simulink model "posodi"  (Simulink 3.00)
settings: Solver=ode45  StartTime=0.0  StopTime=1200  RelTol=1e-3
undefined symbols (not defined in the file or in its folder): dec2bin, H10_X1, H10_X2, H12_X1, H12_X2, H7_X1, H7_X2, H8_X1, H8_X2, sgn
libraries: simulink3 x1

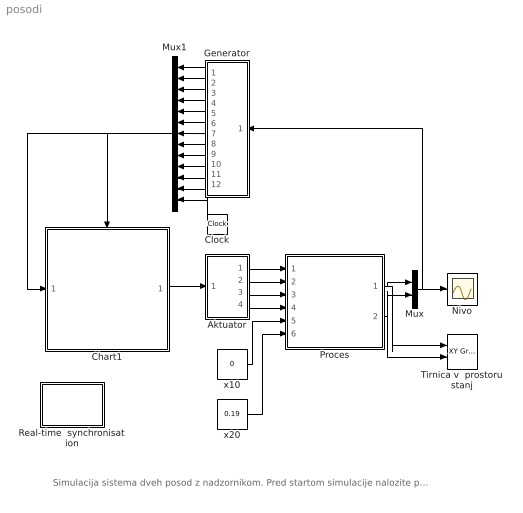
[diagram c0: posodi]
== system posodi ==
  note: Simulacija sistema dveh posod z nadzornikom. Pred startom simulacije nalozite podatke z ukazom "load meje".
  Aktuator : Subsystem
  Chart1 : Stateflow chart
  Clock : Clock
  Generator : Subsystem  Orientation=left
  Mux : Mux  Inputs=2
  Mux1 : Mux  Orientation=left  Inputs=13
  Nivo : Scope
  Proces : Subsystem
  Real-time  synchronisation : Subsystem  mask(Real-time synchronisation){ts=10, tf=20}
      mask prompts: ts "Sample time"; tf "Scale factor"
      mask help: Real-time synchronisation block
  Tirnica v  prostoru stanj : simulink3/Sinks/XY Graph  xmin=0  xmax=1.4  ymin=0  ymax=1.4  st=-1
  x10 : Constant  Value=0
  x20 : Constant  Value=0.19
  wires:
  Aktuator/1(u1) -> Proces/1(u1)
  Aktuator/2(u2) -> Proces/2(u2)
  Aktuator/3(u3) -> Proces/3(u3)
  Aktuator/4(u4) -> Proces/4(u4)
  Chart1/1(u) -> Aktuator/1(us)
  Proces/1(x1) -> Mux/1, Tirnica v  prostoru stanj/1
  Proces/2(x2) -> Mux/2, Tirnica v  prostoru stanj/2
  Mux/1 -> Nivo/1, Generator/1(x)
  Mux1/1 -> Chart1/Trigger, Chart1/1(h)
  x10/1 -> Proces/5(x10)
  x20/1 -> Proces/6(x20)
  Generator/1(h1) -> Mux1/1
  Generator/2(h2) -> Mux1/2
  Generator/3(h3) -> Mux1/3
  Generator/4(h4) -> Mux1/4
  Generator/5(h5) -> Mux1/5
  Generator/6(h6) -> Mux1/6
  Generator/7(h7) -> Mux1/7
  Generator/8(h8) -> Mux1/8
  Generator/9(h9) -> Mux1/9
  Generator/10(h10) -> Mux1/10
  Generator/11(h11) -> Mux1/11
  Generator/12(h12) -> Mux1/12
  Clock/1 -> Mux1/13

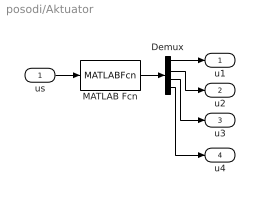
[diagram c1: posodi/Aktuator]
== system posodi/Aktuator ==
  us : Inport  Port=1  PortWidth=-1  SampleTime=-1  DataType=auto
  Demux : Demux  Outputs=4
  MATLAB Fcn : MATLABFcn  MATLABFcn=str2num(dec2bin(u(1)-1,4)')  OutputWidth=-1  OutputSignalType=auto
  u1 : Outport  Port=1
  u2 : Outport  Port=2
  u3 : Outport  Port=3
  u4 : Outport  Port=4
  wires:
  MATLAB Fcn/1 -> Demux/1
  Demux/1 -> u1/1
  Demux/2 -> u2/1
  us/1 -> MATLAB Fcn/1
  Demux/3 -> u3/1
  Demux/4 -> u4/1

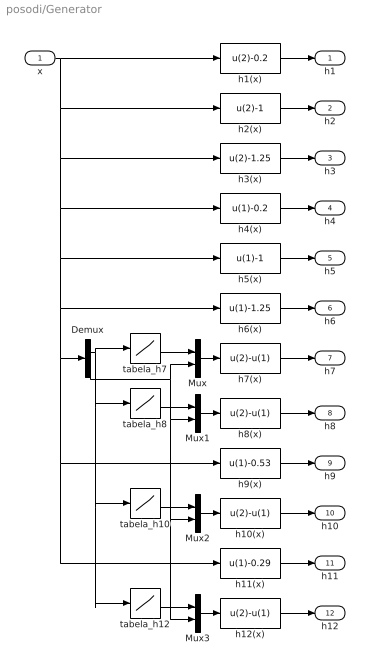
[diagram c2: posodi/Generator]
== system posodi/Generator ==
  x : Inport  Port=1  PortWidth=-1  SampleTime=-1  DataType=auto
  Demux : Demux  Outputs=2
  Mux{,1..3} (4 alike) : Mux  Inputs=2
  h1(x) : Fcn  Expr=u(2)-0.2
  h10(x) : Fcn  Expr=u(2)-u(1)
  h11(x) : Fcn  Expr=u(1)-0.29
  h12(x) : Fcn  Expr=u(2)-u(1)
  h2(x) : Fcn  Expr=u(2)-1
  h3(x) : Fcn  Expr=u(2)-1.25
  h4(x) : Fcn  Expr=u(1)-0.2
  h5(x) : Fcn  Expr=u(1)-1
  h6(x) : Fcn  Expr=u(1)-1.25
  h7(x) : Fcn  Expr=u(2)-u(1)
  h8(x) : Fcn  Expr=u(2)-u(1)
  h9(x) : Fcn  Expr=u(1)-0.53
  tabela_h10 : Lookup  InputValues=H10_X1  OutputValues=H10_X2
  tabela_h12 : Lookup  InputValues=H12_X1  OutputValues=H12_X2
  tabela_h7 : Lookup  InputValues=H7_X1  OutputValues=H7_X2
  tabela_h8 : Lookup  InputValues=H8_X1  OutputValues=H8_X2
  h1 : Outport  Port=1
  h2 : Outport  Port=2
  h3 : Outport  Port=3
  h4 : Outport  Port=4
  h5 : Outport  Port=5
  h6 : Outport  Port=6
  h7 : Outport  Port=7
  h8 : Outport  Port=8
  h9 : Outport  Port=9
  h10 : Outport  Port=10
  h11 : Outport  Port=11
  h12 : Outport  Port=12
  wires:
  x/1 -> h1(x)/1, h2(x)/1, h4(x)/1, h5(x)/1, h9(x)/1, h11(x)/1, Demux/1, h6(x)/1, h3(x)/1
  h1(x)/1 -> h1/1
  h4(x)/1 -> h4/1
  h9(x)/1 -> h9/1
  h11(x)/1 -> h11/1
  Demux/1 -> tabela_h7/1, tabela_h8/1, tabela_h10/1, tabela_h12/1
  tabela_h7/1 -> Mux/1
  Mux/1 -> h7(x)/1
  h7(x)/1 -> h7/1
  Mux1/1 -> h8(x)/1
  h8(x)/1 -> h8/1
  tabela_h8/1 -> Mux1/1
  Mux2/1 -> h10(x)/1
  h10(x)/1 -> h10/1
  Mux3/1 -> h12(x)/1
  h12(x)/1 -> h12/1
  tabela_h10/1 -> Mux2/1
  tabela_h12/1 -> Mux3/1
  h2(x)/1 -> h2/1
  h3(x)/1 -> h3/1
  h5(x)/1 -> h5/1
  h6(x)/1 -> h6/1
  Demux/2 -> Mux1/2, Mux2/2, Mux3/2, Mux/2

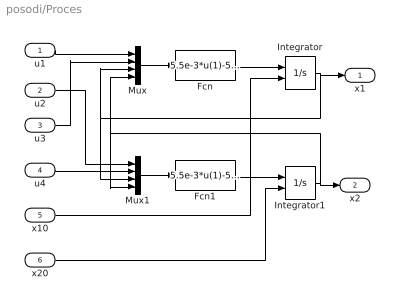
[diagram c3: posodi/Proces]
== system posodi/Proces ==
  u1 : Inport  Port=1  PortWidth=-1  SampleTime=-1  DataType=auto
  u2 : Inport  Port=2  PortWidth=-1  SampleTime=-1  DataType=auto
  u3 : Inport  Port=3  PortWidth=-1  SampleTime=-1  DataType=auto
  u4 : Inport  Port=4  PortWidth=-1  SampleTime=-1  DataType=auto
  x10 : Inport  Port=5  PortWidth=-1  SampleTime=-1  DataType=auto
  x20 : Inport  Port=6  PortWidth=-1  SampleTime=-1  DataType=auto
  Fcn : Fcn  Expr=5.5e-3*u(1)-5e-3*sqrt(u(3))*u(2)-2e-3*sgn(u(3)-u(4))*sqrt(abs(u(3)-u(4)))
  Fcn1 : Fcn  Expr=5.5e-3*u(1)-5e-3*sqrt(u(4))*u(2)+2e-3*sgn(u(3)-u(4))*sqrt(abs(u(3)-u(4)))
  Integrator : Integrator  ExternalReset=none  InitialConditionSource=external  InitialCondition=0.1  LimitOutput=off  UpperSaturationLimit=inf  LowerSaturationLimit=-inf  ShowSaturationPort=off  ShowStatePort=off  AbsoluteTolerance=auto
  Integrator1 : Integrator  ExternalReset=none  InitialConditionSource=external  InitialCondition=0.1  LimitOutput=off  UpperSaturationLimit=inf  LowerSaturationLimit=-inf  ShowSaturationPort=off  ShowStatePort=off  AbsoluteTolerance=auto
  Mux : Mux  Inputs=4
  Mux1 : Mux  Inputs=4
  x1 : Outport  Port=1
  x2 : Outport  Port=2
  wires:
  Mux/1 -> Fcn/1
  Fcn/1 -> Integrator/1
  Integrator/1 -> x1/1, Mux/3, Mux1/3
  Mux1/1 -> Fcn1/1
  Fcn1/1 -> Integrator1/1
  Integrator1/1 -> x2/1, Mux/4, Mux1/4
  u1/1 -> Mux/1
  u3/1 -> Mux/2
  u2/1 -> Mux1/1
  u4/1 -> Mux1/2
  x10/1 -> Integrator/2
  x20/1 -> Integrator1/2

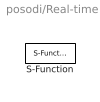
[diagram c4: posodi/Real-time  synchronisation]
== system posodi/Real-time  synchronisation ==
  S-Function : S-Function  FunctionName=rtsinh_f  Parameters=ts,tf  PortCounts=[]  SFunctionModules=''

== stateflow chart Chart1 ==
  state s1/u=10;
  state s8/u=4;
  state s7/u=8;
  state s2a/u=13;
  state s2/u=15;
  state s6/u=7;
  state s3/u=8;
  state s4/u=7;
  state s3a/u=7;
  state s5/u=8;
  (default) -> s8/u=4; : [h[1]>=0&h[3]<0&h[4]<0]
  (default) -> s7/u=8; : [h[4]>=0&h[12]>=0&h[3]<0]
  s8/u=4; -> s1/u=10; : x1
  s7/u=8; -> s8/u=4; : x4
  (default) -> s1/u=10; : [h[1]<0&h[7]<0]
  s1/u=10; -> s2/u=15; : x7
  s6/u=7; -> s7/u=8; : x12
  s2a/u=13; -> s2/u=15; : x7
  (default) -> s2/u=15; : [h[7]>=0&h[5]>=0&h[8]<0&h[6]<0]
  (default) -> s6/u=7; : [h[2]>=0&h[11]<0&h[12]<0]
  (default) -> s2a/u=13; : [h[1]>=0&h[5]>=0&h[7]<0]
  s2/u=15; -> s3/u=8; : x8
  s5/u=8; -> s6/u=7; : x11
  s3a/u=7; -> s3/u=8; : x8
  s3/u=8; -> s4/u=7; : x9
  s4/u=7; -> s5/u=8; : x10
  (default) -> s3/u=8; : [h[8]>=0&h[9]>=0&h[3]<0&h[6]<0]
  (default) -> s4/u=7; : [h[2]>=0&h[9]<0&h[10]<0]
  (default) -> s3a/u=7; : [h[2]>=0&h[8]<0&h[5]<0]
  (default) -> s5/u=8; : [h[10]>=0&h[11]>=0&h[3]<0]
